TYPE ConfigPump :
STRUCT
	LeakRate:SVLREAL;
	
	LeakCheckPumpingTime:SVINT;
	LeakCheckHoldTime:SVINT;
	
	PumpBasePressure:SVINT;
	LeakCheckBasePressur:SVLREAL;
	
	LeakCheckGasLineNums:STRING;
	
	PumpTimeLimit:SVLREAL;
	PumpValveDelay:SVINT;
	
	PumpCrossingPressure:SVINT;
	PumpVHe2FlowPressure:SVINT;
	
	LoadLockPumpBasePressure:SVINT;
	LoadLockPumpTimeLimit:SVINT;
	
	LoadLockPurgeVentPressure:SVINT;
	LoadLockPurgeCycleCount:SVINT;
	LoadLockPurgePumpTime:SVINT;
	
	LoadLockLeakCheckPumpTime:SVINT;
	LoadLockLeakCheckWaitTime:SVINT;
	LoadLockLeakRate:SVLREAL;
END_STRUCT
END_TYPE
